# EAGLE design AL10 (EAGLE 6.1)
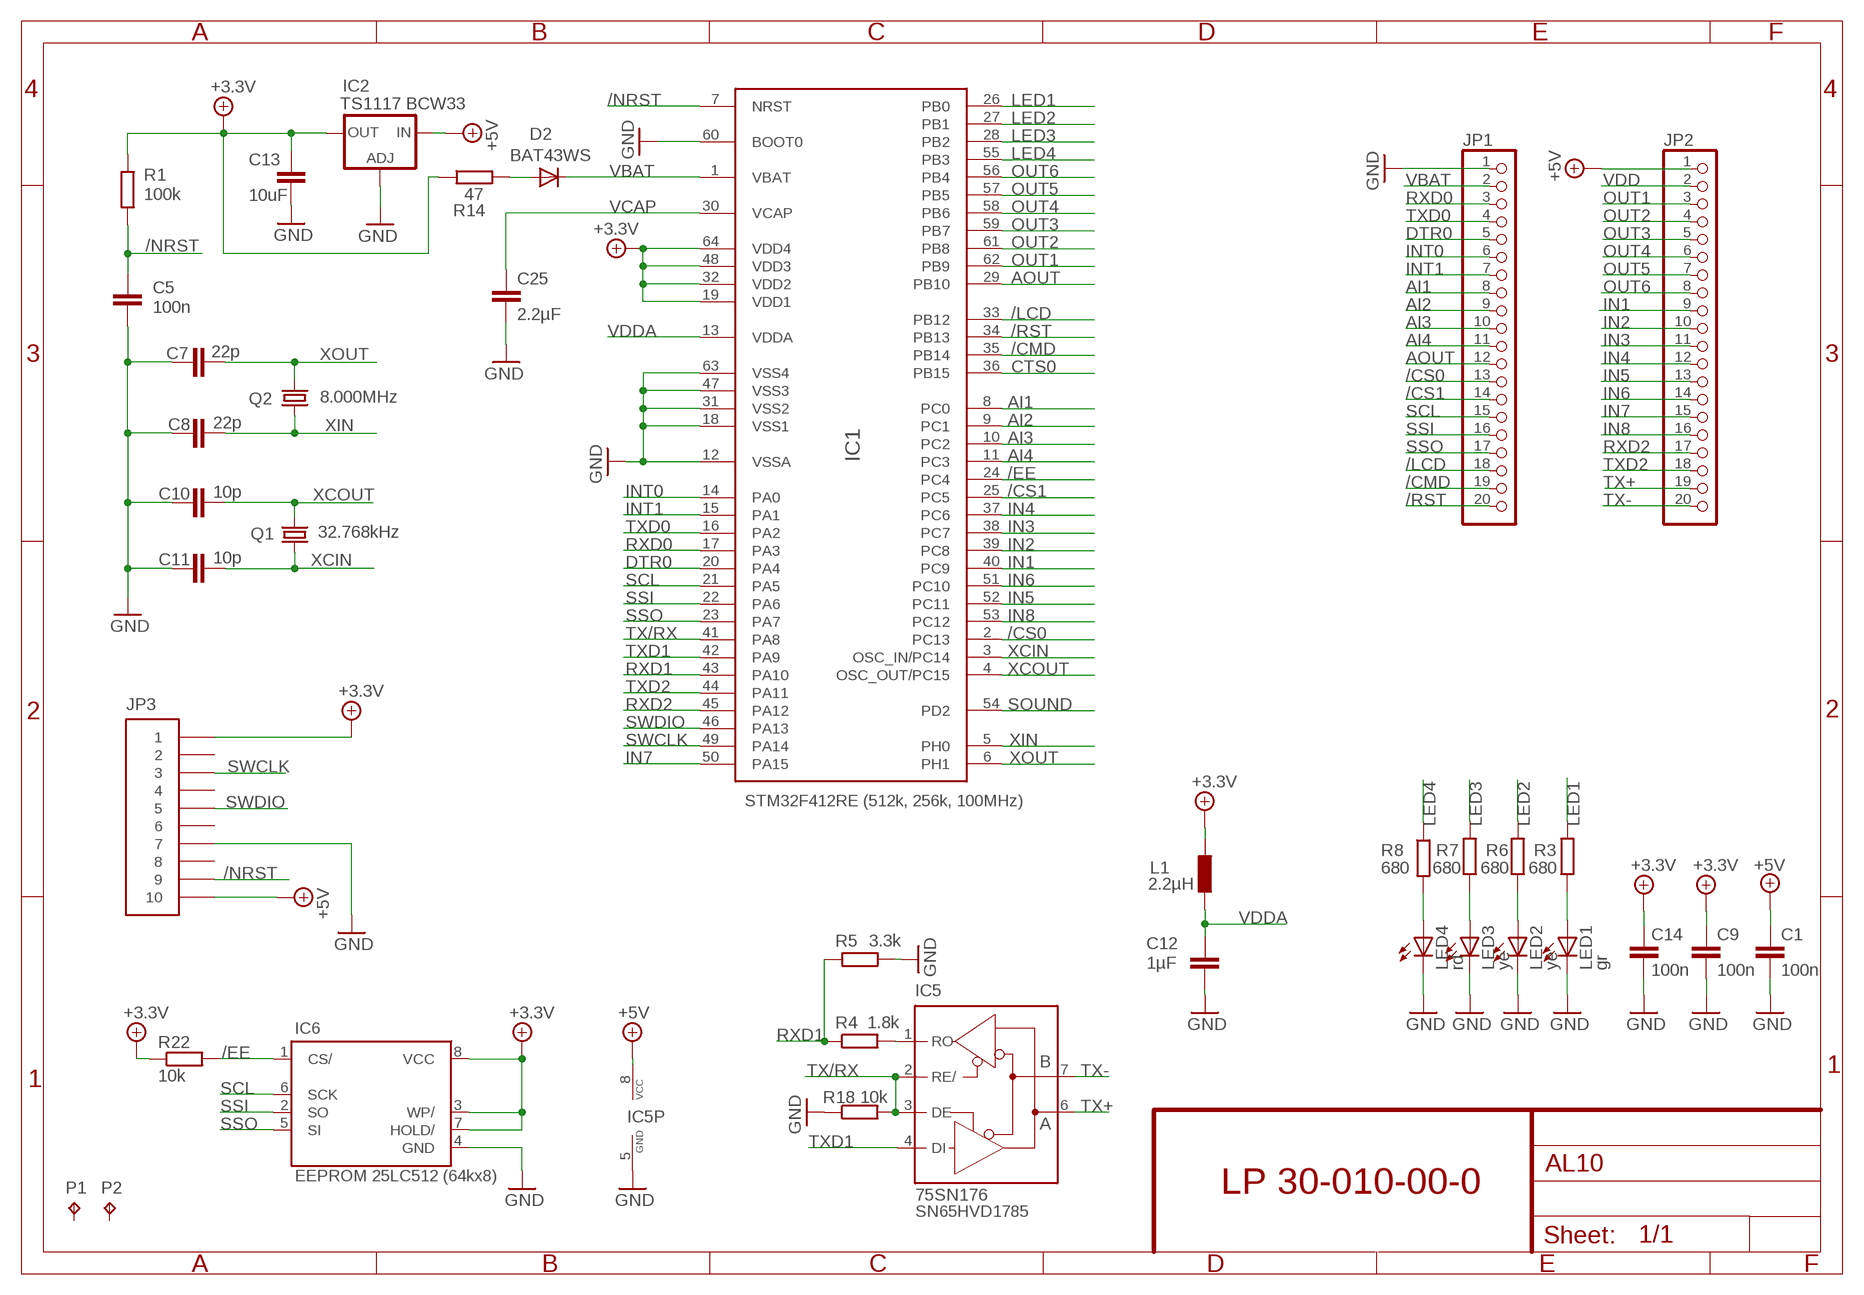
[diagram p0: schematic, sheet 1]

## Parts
C1  100n  C-EUC0603  [C0603]
C5  100n  C-EUC0603  [C0603]
C7  22p  C-EUC0603  [C0603]
C8  22p  C-EUC0603  [C0603]
C9  100n  C-EUC0603  [C0603]
C10  10p  C-EUC0603  [C0603]
C11  10p  C-EUC0603  [C0603]
C12  1µF  C-EUC0603  [C0603]
C13  10uF  C-EUC1206  [C1206]
C14  100n  C-EUC0603  [C0603]
C25  2.2µF  C-EUC1210  [C1210]
D2  BAT43WS  DIODE-SOD323-R  [SOD323-R]
IC1  STM32F412RE  STM32F401XXSTM32F405XX  [LQFP64]
IC2  TS1117 BCW33  LM317MBSTT3  [SOT223]
IC5  75SN176  MAX481CSA  [SO08]
IC6  EEPROM 25LC512 (64kx8)  FM25V20  [SO08]
JP1  CON1X20  [P1X20]
JP2  CON1X20  [P1X20]
JP3  MICROMATCH10  [MICROMATCH10]
L1  2.2µH  R-EU_R0603  [R0603]
LED1  gr  LEDCHIP-LED0805  [CHIP-LED0805]
LED2  ye  LEDCHIP-LED0805  [CHIP-LED0805]
LED3  ye  LEDCHIP-LED0805  [CHIP-LED0805]
LED4  rd  LEDCHIP-LED0805  [CHIP-LED0805]
P1  TPB1,27  [B1,27]
P2  TPB1,27  [B1,27]
Q1  32.768kHz  TF323N32K7680  [TF32]
Q2  8.000MHz  CRYSTALMJ  [MJ]
R1  100k  R-EU_R0603  [R0603]
R3  680  R-EU_R0603  [R0603]
R4  1.8k  R-EU_R0603  [R0603]
R5  3.3k  R-EU_R0603  [R0603]
R6  680  R-EU_R0603  [R0603]
R7  680  R-EU_R0603  [R0603]
R8  680  R-EU_R0603  [R0603]
R14  47  R-EU_R0603  [R0603]
R18  10k  R-EU_R0603  [R0603]
R22  10k  R-EU_R0603  [R0603]

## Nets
+5V: C1.1 IC2.3(IN) IC5.8(VCC) JP2.1 JP3.10
/CMD: IC1.35(PB14) JP1.19
/CS0: IC1.2(PC13) JP1.13
/CS1: IC1.25(PC5) JP1.14
/EE: IC1.24(PC4) IC6.1(CS/) R22.2
/LCD: IC1.33(PB12) JP1.18
/NRST: C5.1 IC1.7(NRST) JP3.9 R1.1
/RST: IC1.34(PB13) JP1.20
AI1: IC1.8(PC0) JP1.8
AI2: IC1.9(PC1) JP1.9
AI3: IC1.10(PC2) JP1.10
AI4: IC1.11(PC3) JP1.11
AOUT: IC1.29(PB10) JP1.12
CTS0: IC1.36(PB15)
DTR0: IC1.20(PA4) JP1.5
GND: C1.2 C5.2 C7.1 C8.1 C9.2 C10.1 C11.1 C12.1 C13.2 C14.1 C25.2 IC1.12(VSSA) IC1.18(VSS1) IC1.31(VSS2) IC1.47(VSS3) IC1.60(BOOT0) IC1.63(VSS4) IC2.1(ADJ) IC5.5(GND) IC6.4(GND) JP1.1 JP3.7 LED1.C LED2.C LED3.C LED4.C R5.1 R18.1
IN1: IC1.40(PC9) JP2.9
IN2: IC1.39(PC8) JP2.10
IN3: IC1.38(PC7) JP2.11
IN4: IC1.37(PC6) JP2.12
IN5: IC1.52(PC11) JP2.13
IN6: IC1.51(PC10) JP2.14
IN7: IC1.50(PA15) JP2.15
IN8: IC1.53(PC12) JP2.16
INT0: IC1.14(PA0) JP1.6
INT1: IC1.15(PA1) JP1.7
LED1: IC1.26(PB0) R3.1
LED2: IC1.27(PB1) R6.1
LED3: IC1.28(PB2) R7.1
LED4: IC1.55(PB3) R8.1
N$1: LED4.A R8.2
N$2: LED3.A R7.2
N$4: LED2.A R6.2
N$5: LED1.A R3.2
N$6: D2.A R14.2
N$26: IC5.1(RO) R4.2
OUT1: IC1.62(PB9) JP2.3
OUT2: IC1.61(PB8) JP2.4
OUT3: IC1.59(PB7) JP2.5
OUT4: IC1.58(PB6) JP2.6
OUT5: IC1.57(PB5) JP2.7
OUT6: IC1.56(PB4) JP2.8
RXD0: IC1.17(PA3) JP1.3
RXD1: IC1.43(PA10) R4.1 R5.2
RXD2: IC1.45(PA12) JP2.17
SCL: IC1.21(PA5) IC6.6(SCK) JP1.15
SOUND: IC1.54(PD2)
SSI: IC1.22(PA6) IC6.2(SO) JP1.16
SSO: IC1.23(PA7) IC6.5(SI) JP1.17
SWCLK: IC1.49(PA14) JP3.3
SWDIO: IC1.46(PA13) JP3.5
TX+: IC5.6(A) JP2.19
TX-: IC5.7(B) JP2.20
TX/RX: IC1.41(PA8) IC5.2(RE/) IC5.3(DE) R18.2
TXD0: IC1.16(PA2) JP1.4
TXD1: IC1.42(PA9) IC5.4(DI)
TXD2: IC1.44(PA11) JP2.18
VBAT: D2.C IC1.1(VBAT) JP1.2
VCAP: C25.1 IC1.30(VCAP)
VDD: C9.1 C13.1 C14.2 IC1.19(VDD1) IC1.32(VDD2) IC1.48(VDD3) IC1.64(VDD4) IC2.4(OUT) IC6.3(WP/) IC6.7(HOLD/) IC6.8(VCC) JP2.2 JP3.1 L1.2 R1.2 R14.1 R22.1 ; supply symbol labelled +3.3V
VDDA: C12.2 IC1.13(VDDA) L1.1
XCIN: C11.2 IC1.3(OSC_IN/PC14) Q1.1
XCOUT: C10.2 IC1.4(OSC_OUT/PC15) Q1.2
XIN: C8.2 IC1.5(PH0) Q2.P1
XOUT: C7.2 IC1.6(PH1) Q2.P3
Unconnected: JP3.2 JP3.4 JP3.6 JP3.8 P1.TP P2.TP Q2.P2(GND) Q2.P4(GND1)

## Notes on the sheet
- STM32F412RE (512k, 256k, 100MHz)
- LP 30-010-00-0
- SN65HVD1785

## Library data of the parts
C1 C5 C7-C14 C25 = rcl:C-EU: CAPACITOR, European symbol
D2 = diode:DIODE-: DIODE
IC1 = stm32f:STM32F401XX: Features • Core: ARM 32-bit Cortex™-M4 CPU with FPU, Adaptive real-time accelerator (ART Accelerator™) allowing 0-wait state execution from Flash memory, frequency up to 84 MHz, memory protection unit, 210 DMIPS/ 1.25 DMIPS/MHz (Dhrystone 2.1), and DSP instructions • Memories – 512kB of Flash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
IC2 = v-reg:LM317?*: 500 mA Adjustable Output Positive Voltage Regulator Source: http://www.onsemi.co.jp .. LM317M-D.PDF
IC5 = maxim:MAX481CSA: RS485 TRANSEIVER; MF: MAXIM; MPN: MAX481CSA; OC_FARNELL: unknown; OC_NEWARK: 90C3817
IC6 = fram:FM25V20: Cypress Ferroelectric RAM 2Mb; MF: Cypress Semiconductor; MOUSER: 877-FM25V20-G; MPN: FM25V20-G
JP1 JP2 = Pins:CON1X20
JP3 = Pins:MICROMATCH10
L1 R1 R3-R8 R14 R18 R22 = rcl:R-EU_: RESISTOR, European symbol
LED1-LED4 = led:LED: LED
P1 P2 = testpad:TP: Test pad
Q1 = tf32:TF32: TF32 Series Tuning Fork Crystal; MF: CTS; MPN: TF323N32K7680; OC_FARNELL: unknown; OC_NEWARK: unknown
Q2 = crystal:CRYSTAL

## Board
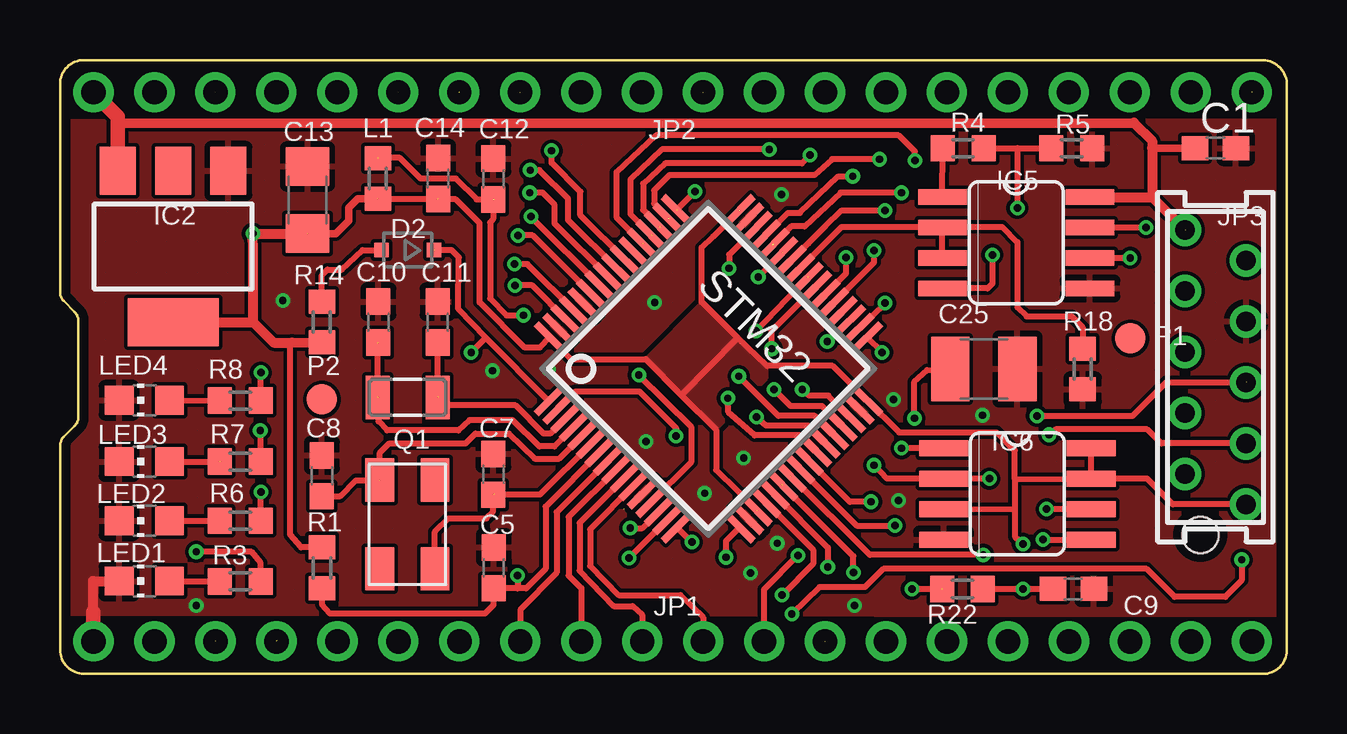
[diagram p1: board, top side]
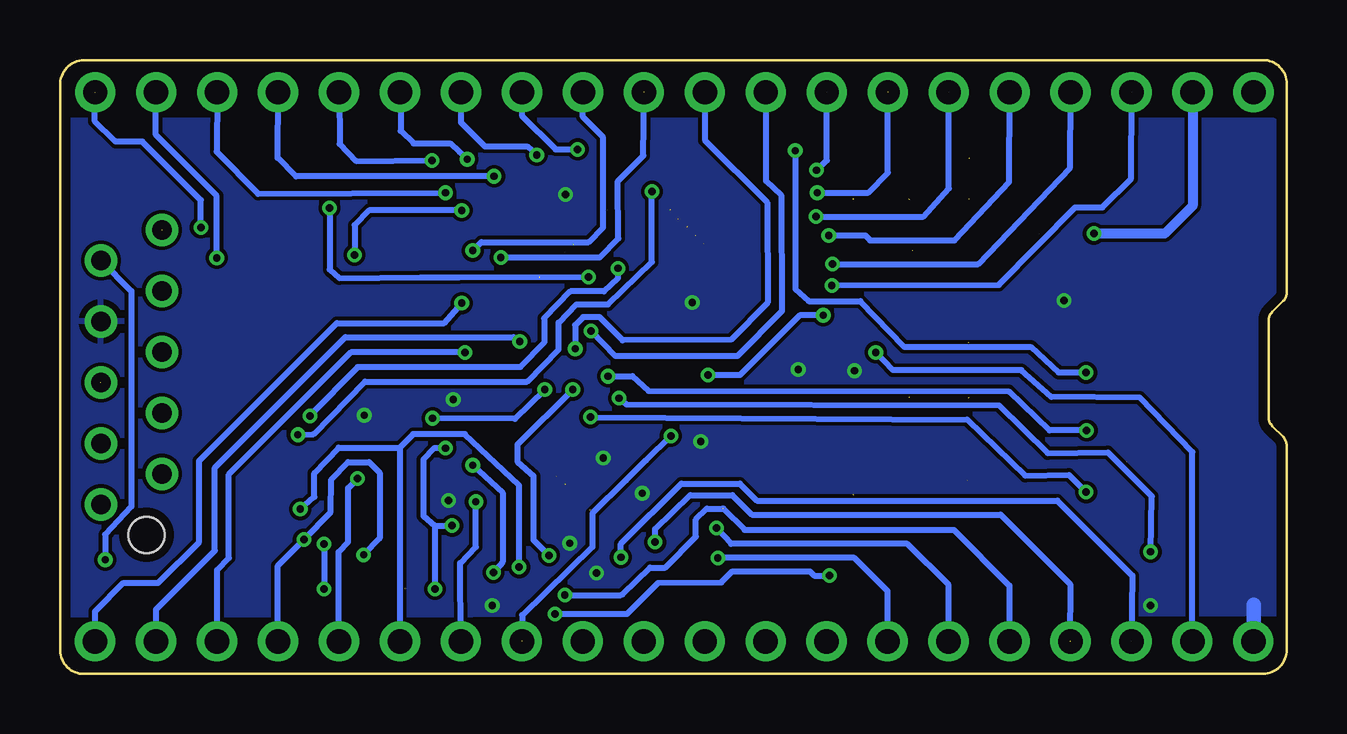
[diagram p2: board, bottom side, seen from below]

Size 51.12 x 25.58 mm. Coordinates in mm from the lower left corner, seen from the top.
Outline: 12.07,0.01 50.12,0 arc93 51.12,1.07 51.12,24.51 arc90 50.12,25.58 1,25.58 arc89 0,24.58 0,15.9 arc45 0.15,15.55 0.6,15.09 arc-45 0.76,14.74 0.76,10.68 arc-45 0.6,10.33 0.16,9.88 arc45 0.01,9.53 0,1.01 arc90 1,0.01 12.16,0
Copper layers (1*16): Top 0.035mm / dielectric 1.5mm / Bottom 0.035mm
Design rules: minimum track width 8mil, minimum drill 12mil, track to track 6mil, track to pad 6mil, pad to pad 6mil, via to via 6mil, smd to smd 6mil, copper to edge 15mil, drill to drill 8mil, minimum pad ring 10mil, minimum via ring 6mil, stop-mask expansion 4mil, vias tented up to drill 0mil, thermal gap 10mil

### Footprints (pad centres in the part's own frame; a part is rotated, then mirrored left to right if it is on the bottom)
C0603 = smd 1.1 x 1: 1 -0.85,0; 2 0.85,0
C1206 = smd 1.6 x 1.8: 1 -1.4,0; 2 1.4,0
C1210 = smd 1.6 x 2.7: 1 -1.4,0; 2 1.4,0
SOD323-R = smd 0.6 x 0.6: A 1.1,0; C -1.1,0
LQFP64 = smd 0.3 x 1.6: 1 -3.75,-5.6; 2 -3.25,-5.6; 3 -2.75,-5.6; 4 -2.25,-5.6; 5 -1.75,-5.6; 6 -1.25,-5.6; 7 -0.75,-5.6; 8 -0.25,-5.6; 9 0.25,-5.6; 10 0.75,-5.6; 11 1.25,-5.6; 12 1.75,-5.6; 13 2.25,-5.6; 14 2.75,-5.6; 15 3.25,-5.6; 16 3.75,-5.6; 33 3.75,5.6; 34 3.25,5.6; 35 2.75,5.6; 36 2.25,5.6; 37 1.75,5.6; 38 1.25,5.6; 39 0.75,5.6; 40 0.25,5.6; 41 -0.25,5.6; 42 -0.75,5.6; 43 -1.25,5.6; 44 -1.75,5.6; 45 -2.25,5.6; 46 -2.75,5.6; 47 -3.25,5.6; 48 -3.75,5.6 | smd 1.6 x 0.3: 17 5.6,-3.75; 18 5.6,-3.25; 19 5.6,-2.75; 20 5.6,-2.25; 21 5.6,-1.75; 22 5.6,-1.25; 23 5.6,-0.75; 24 5.6,-0.25; 25 5.6,0.25; 26 5.6,0.75; 27 5.6,1.25; 28 5.6,1.75; 29 5.6,2.25; 30 5.6,2.75; 31 5.6,3.25; 32 5.6,3.75; 49 -5.6,3.75; 50 -5.6,3.25; 51 -5.6,2.75; 52 -5.6,2.25; 53 -5.6,1.75; 54 -5.6,1.25; 55 -5.6,0.75; 56 -5.6,0.25; 57 -5.6,-0.25; 58 -5.6,-0.75; 59 -5.6,-1.25; 60 -5.6,-1.75; 61 -5.6,-2.25; 62 -5.6,-2.75; 63 -5.6,-3.25; 64 -5.6,-3.75
SOT223 = smd 1.5 x 2: 1 -2.3,-3.15; 2 0,-3.15; 3 2.3,-3.15 | smd 3.8 x 2: 4 0,3.15
SO08 = smd 0.66 x 2.032: 1 -1.905,-3.073; 2 -0.635,-3.073; 3 0.635,-3.073; 4 1.905,-3.073; 5 1.905,3.073; 6 0.635,3.073; 7 -0.635,3.073; 8 -1.905,3.073
P1X20 = drill 1.016 pad 1.676: 1 -24.13,0; 2 -21.59,0; 3 -19.05,0; 4 -16.51,0; 5 -13.97,0; 6 -11.43,0; 7 -8.89,0; 8 -6.35,0; 9 -3.81,0; 10 -1.27,0; 11 1.27,0; 12 3.81,0; 13 6.35,0; 14 8.89,0; 15 11.43,0; 16 13.97,0; 17 16.51,0; 18 19.05,0; 19 21.59,0; 20 24.13,0
MICROMATCH10 = drill 0.813 pad 1.35: 1 -5.715,-1.27; 2 -4.445,1.27; 3 -3.175,-1.27; 4 -1.905,1.27; 5 -0.635,-1.27; 6 0.635,1.27; 7 1.905,-1.27; 8 3.175,1.27; 9 4.445,-1.27; 10 5.715,1.27 | hole 1.5: -6.985,0.635
R0603 = smd 1 x 1.1: 1 -0.85,0; 2 0.85,0
CHIP-LED0805 = smd 1.2 x 1.2: A 0,-1.05; C 0,1.05
B1,27 = smd 1.27 x 1.27: TP 0,0
TF32 = smd 1 x 1.8: 1 -1.25,0; 2 1.25,0
MJ = smd 1.8 x 1.2: P1 -1.85,-1.15; P2 1.85,-1.15; P3 1.85,1.15; P4 -1.85,1.15

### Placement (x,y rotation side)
C1  48.15,21.9 0 top
C5  18.08,4.42 90 top
C7  18.06,8.32 270 top
C8  10.91,8.26 270 top
C9  42.23,3.54 0 top
C10  13.26,14.66 270 top
C11  15.73,14.66 270 top
C12  18.06,20.63 270 top
C13  10.31,19.74 90 top
C14  15.75,20.64 270 top
C25  38.49,12.71 0 top
D2  14.49,17.66 180 top
IC1  27.01,12.72 315 top
IC2  4.71,17.81 180 top
IC5  39.84,17.97 270 top
IC6  39.89,7.5 270 top
JP1  25.53,1.36 0 top
JP2  25.52,24.24 0 top
JP3  48.15,12.78 90 top
L1  13.24,20.64 270 top
LED1  3.51,3.87 90 top
LED2  3.51,6.39 90 top
LED3  3.51,8.85 90 top
LED4  3.51,11.41 90 top
P1  44.6,13.98 0 top
P2  10.91,11.44 0 top
Q1  14.48,11.52 180 top
Q2  14.47,6.23 270 top
R1  10.92,4.42 90 top
R3  7.51,3.86 180 top
R4  37.63,21.9 180 top
R5  42.15,21.9 180 top
R6  7.51,6.39 180 top
R7  7.51,8.85 180 top
R8  7.51,11.39 180 top
R14  10.91,14.67 90 top
R18  42.61,12.71 90 top
R22  37.61,3.54 180 top

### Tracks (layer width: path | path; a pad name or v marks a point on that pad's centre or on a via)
+5V  (1 unrouted)
  Top 0.305: C1.1 45.5,21.9
  Top 0.406: IC5.8 45.5,19.87 | 45.5,19.87 JP3.10 | 2.41,22.95 44.74,22.97 45.5,22.21 45.5,21.9 45.5,19.87
  Top 0.61: IC2.3 2.41,22.95 2.41,23.22 JP2.1
/CMD  (via drill 0.3)
  Top 0.254: v31.97,13.85 IC1.35
  Bottom 0.254: JP1.19 47.12,2.69 44.67,5.14 44.67,8.6 39.23,14.03 32.22,14.03 v31.97,13.85
/CS0  (via drill 0.3)  (1 unrouted)
  Top 0.254: IC1.2 21.47,11.77 24.14,11.77 25.67,10.25 v25.67,9.92
  Bottom 0.254: v25.67,9.92 26.71,8.9 27.55,8.06 28.94,6.69 28.94,5.29 31.87,2.45 31.87,1.36
/CS1  (via drill 0.3)
  Top 0.254: v33.8,7.17 32.91,7.17 IC1.25
  Bottom 0.254: JP1.14 34.44,4.62 33.8,5.29 v33.8,7.17
/EE  (via drill 0.3)  (1 unrouted)
  Top 0.254: IC1.24 33.2,6.18 v34.79,6.18 | v35.5,3.54 36.74,3.54 | IC6.1 v35.07,9.41
  Bottom 0.254: 35.5,6.18 v35.5,3.54 | v35.07,9.41 35.52,9.41 35.98,8.93 35.98,6.59 35.5,6.18 | 35.5,6.18 v34.79,6.18
/LCD  (via drill 0.3)
  Top 0.254: IC1.33 v34.25,13.4
  Bottom 0.254: JP1.18 44.58,4.34 44.08,4.84 44.08,8.32 39,13.4 v34.25,13.4
/NRST  (via drill 0.3)
  Top 0.254: IC1.7 20.23,6.97 20.23,4.38 19.42,3.57 19.06,3.57 | 19.06,3.57 18.09,3.57 C5.1 18.06,3.59 18.07,2.88 17.72,2.52 11.24,2.52 10.91,2.91 R1.1 | v49.24,4.76 49.24,3.9 48.55,3.21 46.44,3.21 45.28,4.38 34.3,4.38 33.54,3.62 31.64,3.62 v30.49,2.5 | v19.06,4.1 19.06,3.57
  Bottom 0.254: JP3.9 48.15,15.96 48.15,6.97 49.24,5.8 v49.24,4.76 | v30.49,2.5 27.5,2.5 26.2,3.79 23.56,3.82 23.1,4.28 19.88,4.28 19.7,4.1 v19.06,4.1
/RST  (via drill 0.3)
  Top 0.254: v34.38,15.45 IC1.34
  Bottom 0.254: JP1.20 49.66,2.61 48.48,3.79 47.03,3.79 45.33,5.5 45.33,8.87 39.59,14.61 35.12,14.61 v34.38,15.45
AI1
  Top 0.254: IC1.8 20.69,6.75 20.69,4.23 19.18,2.67 JP1.8
AI2
  Top 0.254: IC1.9 21.2,6.55 21.2,4.1 21.72,3.58 JP1.9
AI3
  Top 0.254: IC1.10 21.65,6.3 21.65,4.3 23.08,2.83 23.86,2.83 24.26,2.46 JP1.10
AI4
  Top 0.254: IC1.11 22.09,6.02 22.09,4.51 23.28,3.29 25.85,3.29 26.8,2.36 JP1.11
AOUT  (via drill 0.3)
  Top 0.254: JP1.12 29.34,3.53 v30.75,4.94 | IC1.29 31.75,11.16 30.44,11.16 v29.76,11.85
  Bottom 0.254: v30.75,4.94 31.38,5.57 31.38,8.24 32.07,8.85 32.07,9.56 v29.76,11.85
DTR0  (via drill 0.3)  (1 unrouted)
  Top 0.254: IC1.20 31.38,5.17 31.38,4.58 v30.09,3.29
  Bottom 0.254: v30.09,3.29 27.75,3.29 27.67,3.31 26.53,4.43 25.9,4.43 24.63,5.72 24.63,6.44 24.17,6.89 23.51,6.89 | 23.48,6.89 22.59,6 13.88,6 11.56,3.68 JP1.5
GND  (via drill 0.3)
  Top 0.406: 1.39,2.58 1.39,3.85 1.4,3.86 arc45 1.39,3.87 2.45,3.87
  Top 0.61: JP1.1 1.39,1.71 1.39,2.58
  Bottom 0.61: 1.39,1.38 1.39,2.88
  other vias: 26.86,7.53 24.78,15.48 28.49,9 18.02,12.63 28.77,4.2 29.88,5.45 30.06,19.97 20.36,12.68 38.44,10.78 33.11,2.85 9.28,15.55 24.42,9.69 34.73,11.44 34.94,7.22 5.68,2.85
  pour Top (rank 2, hatched): 50.74,23.06 50.71,2.47 0.42,2.52 0.42,9.61 1.13,10.32 1.13,15.02 0.39,15.76 0.39,23.01
  pour Bottom: 0.54,23.04 50.7,23.04 50.7,2.47 0.41,2.53 0.39,9.66 1.11,10.37 1.11,15.02 0.41,15.72 0.41,22.91
IN1  (via drill 0.3)  (1 unrouted)
  Top 0.254: v28.99,14.28 31.15,16.55
  Bottom 0.254: JP2.9 21.71,20.55 21.07,19.95 21.04,15.12 22.9,13.24 27.98,13.24 v28.99,14.28
IN2  (via drill 0.3)
  Top 0.254: v29.66,13.55 29.66,14.3 IC1.39
  Bottom 0.254: JP2.10 24.25,22.24 21.65,19.64 21.64,15.47 23.15,13.93 27.67,13.9 28.64,14.87 29.33,14.87 29.66,14.54 v29.66,13.55
IN3  (via drill 0.3)  (1 unrouted)
  Top 0.254: IC1.38 32.75,16.69 v32.75,17.36
  Bottom 0.254: v32.75,17.36 28.64,17.36 27.85,18.15 27.88,20.53 26.81,21.6 JP2.11
IN4  (via drill 0.3)
  Top 0.254: IC1.37 33.92,17.15 v33.92,17.64
  Bottom 0.254: v33.92,17.64 33.57,17.99 29.1,17.99 28.49,18.6 28.49,22.36 29.33,23.21 JP2.12
IN5  (via drill 0.3)  (1 unrouted)
  Top 0.254: v29.55,21.85 25.08,21.85 23.76,20.61 23.76,19.16 IC1.52
  Bottom 0.254: JP2.13 31.87,23.26 30.47,21.85 v29.55,21.85
IN6  (via drill 0.3)  (1 unrouted)
  Top 0.254: v31.26,21.63 30.93,21.27 25.21,21.27 24.3,20.43 24.3,19.34 24.98,18.65
  Bottom 0.254: JP2.14 34.41,22.98 33.41,21.98 31.66,21.98 v31.26,21.63
IN7  (via drill 0.3)  (1 unrouted)
  Top 0.254: v34.15,21.45 32.17,21.45 31.43,20.79 25.39,20.79 24.75,20.15 24.75,19.59 25.39,18.96
  Bottom 0.254: JP2.15 36.93,22.62 36.39,22.11 34.86,22.11 34.48,21.75 v34.15,21.45
IN8  (via drill 0.3)  (1 unrouted)
  Top 0.254: v35.62,21.4 35.62,21.78 34.94,22.44 24.83,22.44 23.18,20.91 23.18,19.03 IC1.53
  Bottom 0.254: JP2.16 39.47,22.09 38.77,21.37 v35.62,21.4
INT0  (via drill 0.3)
  Top 0.254: v23.76,6.08 24.27,6.08 IC1.14
  Bottom 0.254: JP1.6 14.1,3.71 15.81,5.42 23.15,5.42 v23.76,6.08
INT1  (via drill 0.3)
  Top 0.254: v23.71,4.84 23.73,4.84 IC1.15
  Bottom 0.254: JP1.7 16.64,3.45 18.02,4.84 v23.71,4.84
LED1  (via drill 0.3)
  Top 0.254: R3.1 8.36,4.63 7.99,5.09 v5.68,5.09 | IC1.26 30.85,9.94 28.94,9.94 27.85,10.91 v27.83,11.49
  Bottom 0.254: v5.68,5.09 5.63,7.4 7.46,9.23 9.97,9.2 12,11.19 27.52,11.24 v27.83,11.49
LED2  (via drill 0.3)
  Top 0.254: R6.1 v8.36,7.57 v8.37,7.58 | IC1.27 31.18,10.35 29.43,10.35 v29.02,10.7
  Bottom 0.254: v8.37,7.58 9.08,8.29 10.91,8.26 13.32,10.6 v29.02,10.7
LED3  (via drill 0.3)
  Top 0.254: R7.1 8.36,10.09 v8.34,10.14 | IC1.28 31.45,10.75 29.93,10.75 v28.28,12.41
  Bottom 0.254: v8.34,10.14 9.89,10.14 11.6,11.77 26.61,11.8 27.27,12.41 v28.28,12.41
LED4  (via drill 0.3)
  Top 0.254: R8.1 v8.36,12.55 v8.37,12.56 | IC1.55 21.68,19.11 21.68,20.1 20.49,21.3 v20.49,21.8
  Bottom 0.254: v8.37,12.56 9.51,12.56 10.68,13.62 15.94,13.62 17.77,15.53 19.93,15.53 20.49,16.04 v20.49,21.8
N$1
  Top 0.254: LED4.A R8.2
N$2  (1 unrouted)
  Top 0.254: LED3.A R7.2
N$4
  Top 0.254: LED2.A R6.2
N$5
  Top 0.254: LED1.A R3.2
N$6
  Top 0.254: R14.2 10.91,16.62 11.14,16.85 11.75,16.85 12.61,17.66 13.4,17.66 D2.A
N$26
  Top 0.254: IC5.1 R4.2
OUT1  (via drill 0.3)  (1 unrouted)
  Top 0.254: IC1.62 19.68,16.19 v18.96,16.19
  Bottom 0.254: v18.96,16.19 12,16.22 8.83,19.44 7.68,19.44 6.49,20.63 JP2.3
OUT2  (via drill 0.3)
  Top 0.254: IC1.61 19.47,17.08 v18.94,17.08
  Bottom 0.254: v18.94,17.08 12.87,17.08 9.03,21.09 JP2.4
OUT3  (via drill 0.3)
  Top 0.254: IC1.59 19.69,18.27 v19.09,18.27
  Bottom 0.254: v19.09,18.27 17.56,18.27 17.36,18.07 13.86,18.07 11.57,20.51 JP2.5
OUT4  (via drill 0.3)  (1 unrouted)
  Top 0.254: IC1.58 19.67,19 v19.62,19.06
  Bottom 0.254: v19.62,19.06 15.15,19.06 14.09,20.23 JP2.6
OUT5  (via drill 0.3)  (1 unrouted)
  Top 0.254: IC1.57 20.61,18.76 20.61,19.54 20.1,20.05 v19.57,20.05
  Bottom 0.254: v19.57,20.05 17.44,20.05 16.63,20.89 16.63,24.27
OUT6  (via drill 0.3)  (1 unrouted)
  Top 0.254: IC1.56 21.17,18.91 21.17,19.8 19.98,20.99 v19.6,20.99
  Bottom 0.254: v19.6,20.99 19.17,21.4 JP2.8
RXD0  (via drill 0.3)  (1 unrouted)
  Top 0.254: IC1.17 27.75,5.53 v27.75,4.86
  Bottom 0.254: v27.75,4.86 27.75,5.42 25.24,7.93 22.8,7.93 22.09,7.22 9.56,7.22 6.44,4.1 JP1.3
RXD1  (via drill 0.3)  (1 unrouted)
  Top 0.254: 39.89,21.9 R5.2 | R4.1 39.89,21.9 | 39.89,21.9 v39.89,19.42 | v29.1,16.55 IC1.43
  Bottom 0.254: v39.89,19.42 39.89,16.85 39.49,16.49 36.11,16.52 34.51,16.52 v29.1,16.55
RXD2  (via drill 0.3)
  Top 0.254: IC1.45 30.33,19.21 30.82,19.21 32.43,20.74 v33.03,20.74
  Bottom 0.254: v33.03,20.74 41.29,20.74 42.05,21.5 JP2.17
SCL  (via drill 0.3)
  Top 0.254: IC6.6 v41.11,6.87 | IC1.21 31.99,5.26 v31.99,4.45
  Bottom 0.254: v41.11,6.87 40.53,7.38 40.53,8.37 39.51,9.43 36.97,9.43 | 36.97,9.43 36.96,8.36 JP1.15 | v31.99,4.45 31.99,7.86 34.25,9.99 36.41,9.99 36.97,9.43
SSI  (via drill 0.3)  (1 unrouted)
  Top 0.254: v38.72,8.14 IC6.2 34.46,8.14 v33.92,8.7 | v33.06,4.23 33.06,4.91 30.06,7.91
  Bottom 0.254: JP1.16 39.51,5.09 39.12,5.51 39.12,7.74 v38.72,8.14 | v33.92,8.7 32.68,7.55 32.68,4.66 v33.06,4.23 33.11,4.05
SSO  (via drill 0.3)  (1 unrouted)
  Top 0.254: v40.96,5.6 IC6.5 | v38.47,4.96 33.74,4.96 30.44,8.24
  Bottom 0.254: JP1.17 42.04,4.52 v40.96,5.6 39.84,6.74 39.82,8.11 39.13,8.82 38.24,8.82 37.81,8.39 37.81,5.65 v38.47,4.96
SWCLK  (via drill 0.3)  (1 unrouted)
  Top 0.254: JP3.3 45.89,9.61 45.3,10.2 41.49,10.2 v41.21,9.97 | v26.45,20.1 25.69,19.34
  Bottom 0.254: v41.21,9.97 40.55,9.99 38.42,12.18 31.66,12.18 30.34,13.52 30.34,14.64 29.6,15.4 28.28,15.4 26.45,17.15 v26.45,20.1
SWDIO  (via drill 0.3)  (1 unrouted)
  Top 0.254: IC1.46 27.88,17.47 v27.88,16.9 | v40.7,10.75 44.69,10.75 46.09,12.15 49.44,12.15
  Bottom 0.254: v27.88,16.9 27.88,16.49 28.46,15.94 29.86,15.94 30.95,14.82 30.95,13.8 31.94,12.79 38.72,12.79 40.7,10.78 v40.7,10.75
TX+  (via drill 0.3)
  Top 0.254: IC5.6 v44.59,17.33
  Bottom 0.254: v44.59,17.33 44.59,19.92 47.13,22.46 47.13,24.22 JP2.19
TX-  (via drill 0.3)  (1 unrouted)
  Top 0.254: IC5.7 v45.25,18.6
  Bottom 0.254: v45.25,18.6 45.25,19.75 47.69,22.18 48.81,22.18 48.86,22.23 49.67,23.02 49.67,24.24 49.7,24.24
TX/RX
  Top 0.254: IC5.2 IC5.3 36.77,18.63 | IC1.41 32.57,18.63 36.77,18.63 | 36.77,18.63 39.26,18.63 39.89,17.99 39.89,15.28 40.27,14.89 42.15,14.89 42.61,14.44 R18.2
TXD0  (via drill 0.3)  (1 unrouted)
  Top 0.254: IC1.16 v26.33,5.5
  Bottom 0.254: v26.33,5.5 26.33,6.03 24.85,7.45 23.1,7.45 22.29,6.64 11.93,6.64 9.03,3.74 9.06,1.38
TXD1  (via drill 0.3)
  Top 0.254: IC1.42 31.18,17.94 31.89,18.66 32.57,19.31 v34.38,19.31 | v38.85,17.46 38.85,16.27 38.65,16.06 IC5.4
  Bottom 0.254: v34.38,19.31 38.24,19.31 38.85,18.7 v38.85,17.46
TXD2  (via drill 0.3)  (1 unrouted)
  Top 0.254: v35.07,20.05 32.53,20.05 31.03,18.65 30.47,18.65 29.71,17.89
  Bottom 0.254: JP2.18 44.6,21.76 42.86,20 v35.07,20.05
VBAT  (via drill 0.3)  (1 unrouted)
  Top 0.254: IC1.1 20.37,11.36 17.74,14.01 | 17.74,14.01 16.6,15.2 16.63,17.36 16.32,17.66 15.61,17.66 | v17.13,13.4 17.74,14.01
  Bottom 0.254: JP1.2 3.94,9.24 6.13,11.52 9.82,11.54 11.06,12.66 16.42,12.66 v17.13,13.4
VCAP  (via drill 0.3)
  Top 0.254: IC1.30 32.02,11.59 31.21,11.59 30.98,11.83 v30.93,11.85 | v35.6,10.65 35.6,12.18 36.13,12.66 C25.1
  Bottom 0.254: v30.93,11.85 32.17,10.63 v35.6,10.65
VDD  (via drill 0.3)  (5 unrouted)
  Top 0.254: IC6.7 IC6.8 | C9.1 v40.12,3.54 R22.1 38.44,3.6 | L1.2 C14.2 | R1.2 10.04,5.27 9.59,5.8 9.59,13.79 9.66,13.81 | JP3.1 46.37,7.07 45.3,8.14 IC6.7 | IC6.3 39.79,6.89 | 39.79,8.11 IC6.7 | 39.79,8.11 39.79,6.89 | 39.79,6.89 39.79,5.72 v40.12,5.42 | 25.9,11.62 24.4,13.12 21.31,13.12 IC1.64 19.99,13.6 19.37,13.6 17.49,15.48 17.49,18.78 16.5,19.77 15.71,19.77 15.69,19.8 | 29.05,6.82 27.34,8.49 27.34,10.17 25.9,11.62 | 28.23,14.01 26.73,15.5 26.73,17.76 27.22,18.22 28.31,19.31 | 28.23,14.01 29.48,12.84 32.2,12.84 IC1.32 34.97,10.07 39.03,10.07 39.79,9.31 39.79,8.11 | 28.23,14.01 25.9,11.62
  Top 0.305: C13.1 11.49,18.34 12.03,18.88 12.03,19.42 12.41,19.8 L1.2
  Top 0.406: IC2.4 8.05,14.66 | 8.05,14.66 8.9,13.8 9.66,13.81 R14.1 | 8.05,14.66 8.05,17.59 v8.04,18.35 10.33,18.35
  Bottom 0.254: v40.12,5.42 v40.12,3.54
  Bottom 0.406: JP2.2 3.93,19.51 5.09,18.35 v8.04,18.35
  pour Top: 24.45,13.09 26.78,15.45 29.38,12.86 29.38,12.33 27.34,10.27
VDDA  (via drill 0.3)  (2 unrouted)
  Top 0.254: C12.2 18.05,18.96 17.92,18.81 17.92,15.65 18.61,14.95 v19.32,14.95 | v24.12,12.46 26.3,10.3 26.3,8.82 IC1.13 | L1.1 14.16,21.5 15.02,20.63 16.5,20.63 17.36,19.77 18.1,19.77
  Bottom 0.254: v19.32,14.95 20.31,14.95 22.8,12.46 v24.12,12.46
XCIN  (1 unrouted)
  Top 0.254: Q1.1 C11.2 | IC1.3 20.42,10.02 20.16,10.02 18.99,11.19 15.76,11.19 15.76,11.54
XCOUT  (2 unrouted)
  Top 0.254: Q1.2 13.25,13.8 | IC1.4 20.6,9.48 19.98,9.48 18.86,10.58 17.06,10.58 16.6,10.14 13.63,10.14 13.27,10.53 13.27,11.52
XIN  (1 unrouted)
  Top 0.254: C8.2 11.68,7.41 12.33,8.06 13.32,8.06 | Q2.P1 13.33,9.21 13.73,9.61 16.9,9.61 17.31,10.02 18.71,10.02 19.77,8.98 20.8,8.98 IC1.5
XOUT  (1 unrouted)
  Top 0.254: Q2.P3 15.63,5.92 16.19,6.49 17.77,6.49 18.05,6.77 18.1,7.48 | IC1.6 20,7.47 C7.2

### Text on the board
Document: BRICK16
tDocu: LP 30-010-00-0
bDocu: +5V | 3V3 | IN0 | IN1 | IN2 | IN3 | IN4 | IN5 | IN6 | IN7 | RX2 | TX2 | TX+ | TX- | OUT0 | OUT1 | OUT2 | OUT3 | OUT4 | OUT5 | GND | BAT | RXD | TXD | DTR | INT0 | INT1 | AI0 | AI1 | AI2 | AI3 | AO0 | CS0 | CS1 | SCL | SSI | SSO | LCD | CMD | RST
